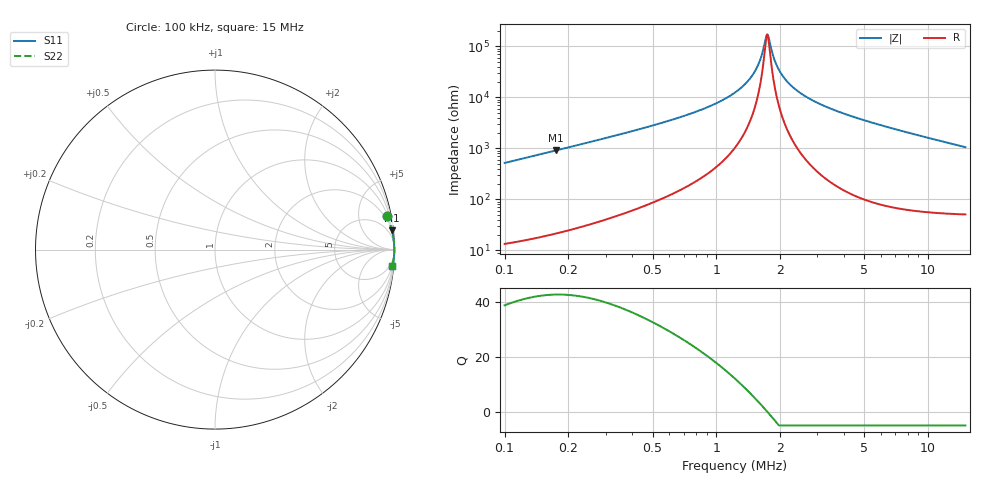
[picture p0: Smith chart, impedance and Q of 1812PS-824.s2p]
# MHz S MA R 50
!Freq  MagS11  AngS11  MagS21  AngS21  MagS12  AngS12  MagS22  AngS22
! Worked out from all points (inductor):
!   801 points, 100 kHz to 15 MHz, reference 50 ohm
!   read as one part in series: L = 820 uH near 102.5 kHz
!   highest Q = 42.7 at 174.6 kHz (marker M1), where L = 828 uH
!   self-resonance near 1.739 MHz
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0.1  0.9771 10.9  0.189 -77.6  0.189 -77.6  0.9771 10.9
0.1746185  0.9915 6.3  0.1091 -82.4  0.1091 -82.4  0.9915 6.3
0.2900143  0.9963 3.7  0.06483 -84.9  0.06483 -84.9  0.9963 3.7
0.4524259  0.998 2.3  0.03993 -86.0  0.03993 -86.0  0.998 2.3
1.150388  0.9993 0.5  0.009516 -85.3  0.009516 -85.3  0.9993 0.5
1.396909  0.9994 0.3  0.004978 -82.5  0.004978 -82.5  0.9994 0.3
1.563616  0.9994 0.1  0.002465 -75.7  0.002465 -75.7  0.9994 0.1
1.623494  0.9994 0.1  0.00166 -68.9  0.00166 -68.9  0.9994 0.1
1.706914  0.9994 0.0  0.0007272 -36.4  0.0007272 -36.4  0.9994 0.0
1.73929  0.9994 0.0  0.0005823 -1.2  0.0005823 -1.2  0.9994 0.0
1.77228  0.9994 -0.0  0.0007074 35.0  0.0007074 35.0  0.9994 -0.0
1.851711  0.9994 -0.1  0.001498 67.5  0.001498 67.5  0.9994 -0.1
1.910617  0.9994 -0.1  0.002161 74.6  0.002161 74.6  0.9994 -0.1
2.046892  0.9994 -0.2  0.003676 81.0  0.003676 81.0  0.9994 -0.2
2.276863  0.9994 -0.3  0.006088 84.4  0.006088 84.4  0.9994 -0.3
2.596924  0.9994 -0.5  0.009179 86.0  0.009179 86.0  0.9994 -0.5
3.551935  0.9992 -1.0  0.01729 87.0  0.01729 87.0  0.9992 -1.0
5.075882  0.9988 -1.6  0.02867 86.8  0.02867 86.8  0.9988 -1.6
7.578772  0.9976 -2.6  0.04589 85.7  0.04589 85.7  0.9976 -2.6
10.04625  0.9959 -3.6  0.06217 84.4  0.06217 84.4  0.9959 -3.6
12.58717  0.9937 -4.5  0.07857 83.1  0.07857 83.1  0.9937 -4.5
15  0.9911 -5.4  0.0939 81.9  0.0939 81.9  0.9911 -5.4
